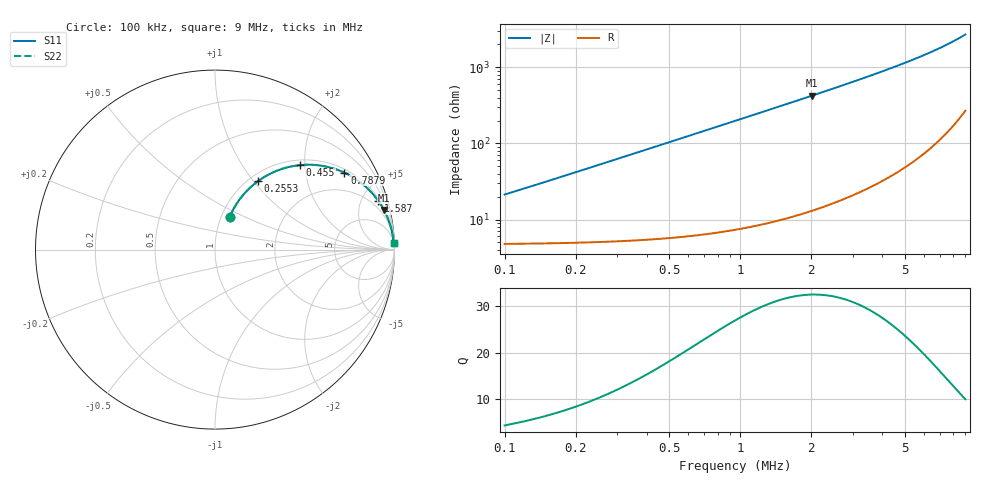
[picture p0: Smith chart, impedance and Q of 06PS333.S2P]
! Coilcraft 0603PS-333 Power Chip Inductor
! 19 February 2003
# MHZ S MA R 50
!Freq  MagS11  AngS11  MagS21  AngS21  MagS12  AngS12  MagS22  AngS22
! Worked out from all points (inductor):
!   403 points, 100 kHz to 9 MHz, reference 50 ohm
!   read as one part in series: L = 33 uH near 144.4 kHz
!   highest Q = 32.6 at 2.008 MHz (marker M1), where L = 33.5 uH
!   S11 on the Smith chart (normalised r, x): 100 kHz: 1.10, +0.41; 255.3 kHz: 1.10, +1.06; 455 kHz: 1.11, +1.89; 787.9 kHz: 1.13, +3.27; 1.587 MHz: 1.21, +6.64; 9 MHz: 6, +54
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0.1  0.1992 65.8  0.9362 -11.2  0.9362 -11.2  0.1992 65.8
0.12219  0.2392 65.7  0.9274 -13.6  0.9274 -13.6  0.2392 65.7
0.18876  0.3523 62.4  0.8929 -20.5  0.8929 -20.5  0.3523 62.4
0.25533  0.4521 57.8  0.8499 -26.7  0.8499 -26.7  0.4521 57.8
0.29971  0.5106 54.7  0.8186 -30.6  0.8186 -30.6  0.5106 54.7
0.34409  0.5627 51.6  0.7862 -34.1  0.7862 -34.1  0.5627 51.6
0.45504  0.6678 44.8  0.706 -41.8  0.706 -41.8  0.6678 44.8
0.61037  0.7678 37.2  0.6052 -50.1  0.6052 -50.1  0.7678 37.2
0.69913  0.8075 33.7  0.5556 -53.8  0.5556 -53.8  0.8075 33.7
0.78789  0.8385 30.7  0.5117 -56.9  0.5117 -56.9  0.8385 30.7
0.94322  0.878 26.5  0.4472 -61.3  0.4472 -61.3  0.878 26.5
1.12074  0.908 22.9  0.3887 -65.2  0.3887 -65.2  0.908 22.9
1.34264  0.9324 19.4  0.3325 -68.7  0.3325 -68.7  0.9324 19.4
1.58673  0.9494 16.6  0.2857 -71.6  0.2857 -71.6  0.9494 16.6
2.00834  0.9666 13.2  0.2285 -75.0  0.2285 -75.0  0.9666 13.2
2.49652  0.9772 10.6  0.1842 -77.6  0.1842 -77.6  0.9772 10.6
3.07346  0.984 8.6  0.1488 -79.6  0.1488 -79.6  0.984 8.6
3.76135  0.9886 6.9  0.1198 -81.1  0.1198 -81.1  0.9886 6.9
4.56019  0.9915 5.5  0.09646 -82.2  0.09646 -82.2  0.9915 5.5
6.04692  0.9942 3.9  0.06815 -83.2  0.06815 -83.2  0.9942 3.9
7.53365  0.9953 2.9  0.04986 -83.1  0.04986 -83.1  0.9953 2.9
9  0.9957 2.1  0.03688 -82.2  0.03688 -82.2  0.9957 2.1
